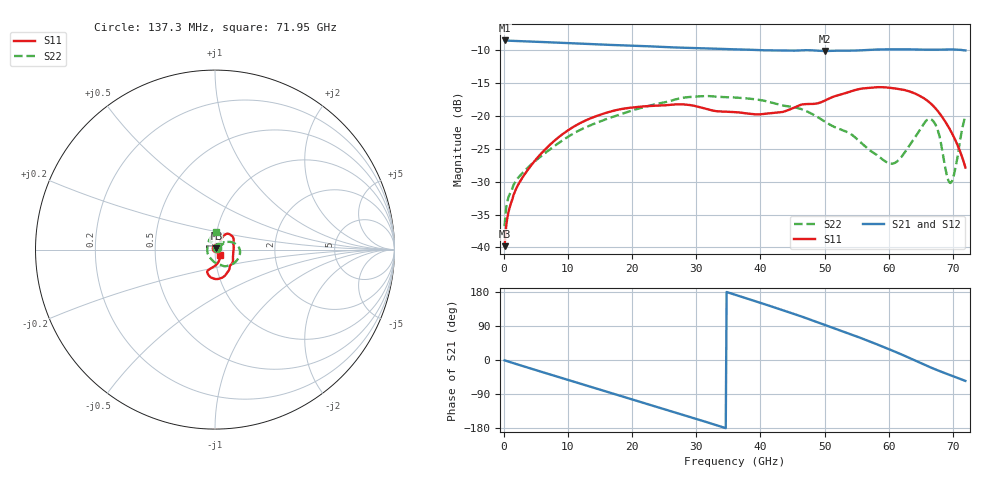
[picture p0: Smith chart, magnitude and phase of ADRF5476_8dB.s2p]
! Device:  ADRF5476
! Description: Flip-Chip, Silicon Digital Step Attenuator
! Frequency:  0.1 GHz -  72 GHz
! Ports:
!  RFC = ATTIN
!  RF1 = ATTOUT
! VDD  =  +3.3 Volts
! VSS  =  -3.3 Volts
! State
! 8dB Attenuation State: D0 = 0V, D1 = +3.3V
! Data:  Data was collected using a calibrated network analyzer
!  The reference plane is the package boundry of ADRF5476 switch.
! Notes: Analog Devices supplies this data as a sample of measured data
!  for this product.  Your particular data for this product may vary.
!  Analog Devices reserves the right to change this data at anytime.
# GHZ  S  DB  R  50
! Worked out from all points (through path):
!   524 points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, 137.3 MHz to 71.95 GHz, reference 50 ohm
!   highest |S21| = -8.58 dB at 137.3 MHz (marker M1); lowest = -10.2 dB at 50.12 GHz (marker M2)
!   group delay of S21, straight-line fit = 15.7 ps
!   lowest |S11| = -39.8 dB at 137.3 MHz (marker M3), VSWR 1.02, Z = 50.8 + j0.665 ohm
!   |S11| at or under -10 dB: start of sweep to end of sweep
!   |S22| runs from -36.8 to -17.0 dB; largest |S21 - S12| = 0.035
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0.1373092  -39.81 39.8  -8.58 -0.9  -8.58 -0.9  -36.77 29.2
0.6865458  -34.90 42.8  -8.61 -3.9  -8.61 -3.9  -32.55 25.3
1.098473  -33.36 43.1  -8.63 -6.1  -8.63 -6.1  -31.53 25.8
3.020802  -29.24 48.5  -8.70 -16.3  -8.70 -16.3  -28.59 30.1
7.277386  -24.34 58.5  -8.86 -38.4  -8.86 -38.4  -25.06 36.2
12.22052  -20.97 58.1  -9.07 -63.9  -9.07 -63.9  -22.01 32.6
17.9875  -19.06 52.5  -9.31 -93.6  -9.31 -93.6  -19.85 23.9
24.16641  -18.48 43.7  -9.54 -125.3  -9.53 -125.3  -18.14 11.7
30.48263  -18.69 26.5  -9.74 -157.9  -9.74 -157.9  -17.05 -5.4
36.11231  -19.46 9.8  -9.92 172.0  -9.92 172.1  -17.24 -21.8
42.0166  -19.58 -15.5  -10.09 139.7  -10.07 139.6  -18.08 -40.3
48.05821  -18.22 -45.6  -10.08 104.6  -10.08 104.6  -19.74 -62.6
50.11784  -17.67 -51.2  -10.18 92.1  -10.17 92.1  -20.94 -70.2
55.19828  -16.00 -72.1  -10.10 61.0  -10.09 60.9  -23.68 -98.2
60.0041  -15.75 -90.3  -9.93 28.7  -9.92 28.7  -27.20 -169.7
61.65181  -15.96 -95.7  -9.91 17.1  -9.91 17.1  -26.62 155.0
66.45763  -18.07 -109.2  -9.99 -19.0  -9.99 -19.2  -20.52 83.2
67.69342  -19.35 -102.6  -9.98 -27.7  -9.98 -28.7  -22.34 54.0
69.06651  -21.30 -86.4  -9.94 -36.6  -9.94 -39.3  -29.08 67.3
69.61574  -22.22 -79.3  -9.94 -40.2  -9.94 -43.6  -30.21 82.2
70.16498  -23.26 -72.3  -9.95 -43.7  -9.95 -47.8  -28.98 97.0
71.95  -27.87 -49.3  -10.09 -55.1  -10.09 -61.6  -19.95 85.6
